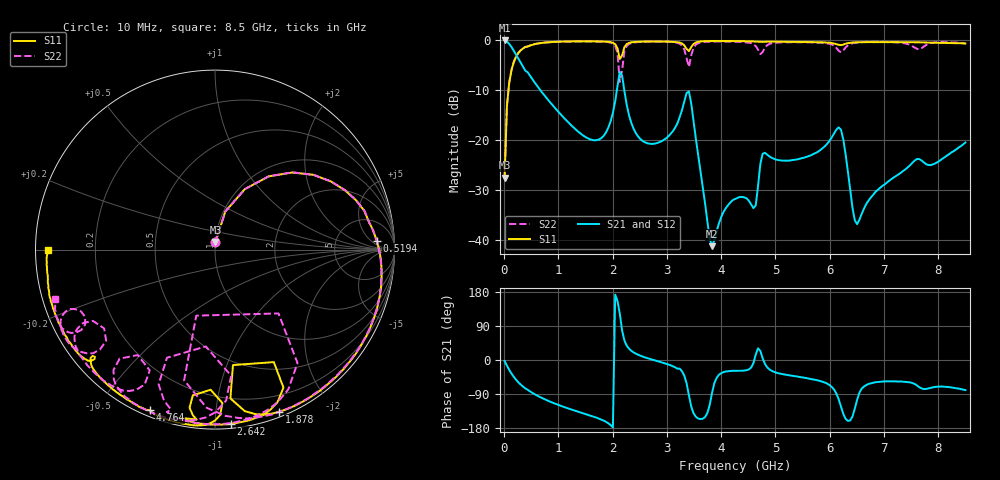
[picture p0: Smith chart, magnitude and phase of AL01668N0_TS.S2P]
!AVX CORPORATION
!PART NUMBER AL01668N0_TS
!DESCRIPTION: AIR CORE INDUCTOR, 68nH, 7 TURNS
!Agilent Technologies,E5071C,MY46102230,A.09.54
!Date: Mon Sep 03 16:35:59 2012
!Data & Calibration Information:
!Freq	S11:SOLT2(ON)	S21:SOLT2(ON)	S12:SOLT2(ON)	S22:SOLT2(ON)
# Hz S dB R 50
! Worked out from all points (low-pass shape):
!   201 points, 10 MHz to 8.5 GHz, reference 50 ohm
!   highest |S21| = -0.01 dB at 10 MHz (marker M1); lowest = -41.3 dB at 3.83 GHz (marker M2)
!   |S21| within 3 dB of the highest: start of sweep to 229.1 MHz
!   lowest |S11| = -27.5 dB at 10 MHz (marker M3), VSWR 1.09, Z = 50.1 + j4.2 ohm
!   |S11| at or under -10 dB: start of sweep to 81.33 MHz
!   |S22| runs from -27.5 to -0.2 dB; largest |S21 - S12| = 0.019
!   S11 on the Smith chart (normalised r, x): 10 MHz: 1.00, +0.08; 519.4 MHz: 15, +8; 1.878 GHz: 0.05, -1.47; 2.642 GHz: 0.03, -1.10; 4.764 GHz: 0.03, -0.67; 8.5 GHz: 0.04, -0.00
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1e7  -27.54 86.3  -0.01 -2.9  -0.14 -2.1  -27.49 86.8
5.245e7  -13.18 74.9  -0.23 -14.8  -0.19 -14.8  -13.14 74.9
1.3735e8  -5.93 53.8  -1.34 -35.9  -1.32 -35.9  -5.90 53.7
5.194e8  -0.89 3.0  -7.76 -86.5  -7.75 -86.6  -0.87 2.5
1.4533e9  -0.19 -50.2  -19.05 -140.5  -19.05 -140.5  -0.21 -53.8
1.8778e9  -0.26 -68.5  -18.47 -163.2  -18.48 -163.2  -0.31 -75.4
2.0476e9  -0.77 -79.6  -12.20 172.6  -12.20 172.6  -1.09 -93.0
2.1325e9  -3.73 -81.2  -6.30 121.9  -6.30 121.9  -8.35 -105.8
2.2174e9  -1.33 -63.6  -10.18 51.4  -10.18 51.4  -2.15 -54.0
2.6419e9  -0.23 -84.7  -20.65 4.8  -20.65 4.8  -0.25 -86.4
2.85415e9  -0.22 -91.0  -20.46 -4.1  -20.44 -4.0  -0.24 -93.6
3.3211e9  -0.99 -99.1  -12.24 -41.4  -12.23 -41.5  -1.79 -112.7
3.406e9  -2.14 -91.8  -10.25 -93.1  -10.25 -93.2  -5.32 -95.4
3.8305e9  -0.12 -97.3  -41.29 -87.9  -41.27 -88.5  -0.23 -104.3
4.255e9  -0.13 -104.1  -31.84 -28.4  -31.85 -28.5  -0.27 -116.1
4.63705e9  -0.22 -110.5  -33.11 14.3  -33.10 14.0  -1.14 -130.1
4.7644e9  -0.30 -112.1  -22.74 4.7  -22.76 4.6  -2.33 -118.4
5.6983e9  -0.35 -129.6  -22.79 -51.1  -22.80 -51.3  -0.40 -141.2
6.2077e9  -0.95 -138.2  -17.92 -123.1  -17.94 -123.2  -2.41 -144.6
6.50485e9  -0.38 -143.0  -36.86 -105.1  -36.96 -105.1  -0.43 -144.2
7.09915e9  -0.34 -154.8  -28.17 -56.4  -28.15 -56.2  -0.31 -152.6
8.5e9  -0.61 -179.8  -20.48 -79.4  -20.49 -79.5  -0.61 -162.8
